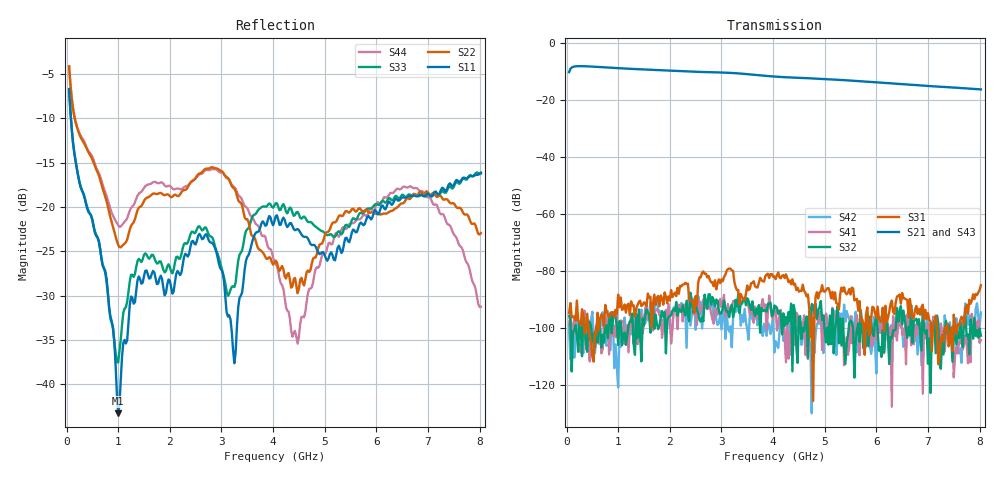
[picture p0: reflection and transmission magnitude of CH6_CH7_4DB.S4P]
!Agilent Technologies,E5071C,MY46316741,A.11.02
!Date: Mon Jun 01 10:34:16 2026
!Data & Calibration Information:
!1:CH6 INPUT 2:CH6 OUTPUT 3:CH7 INPUT 4:CH7 OUTPUT
!Freq	S11:SOLT4(ON)	S12:SOLT4(ON)	S13:SOLT4(ON)	S14:SOLT4(ON)
!	S21:SOLT4(ON)	S22:SOLT4(ON)	S23:SOLT4(ON)	S24:SOLT4(ON)
!	S31:SOLT4(ON)	S32:SOLT4(ON)	S33:SOLT4(ON)	S34:SOLT4(ON)
!	S41:SOLT4(ON)	S42:SOLT4(ON)	S43:SOLT4(ON)	S44:SOLT4(ON)
!PortZ  Port1:50+j0  Port2:50+j0  Port3:50+j0  Port4:50+j0
!Above PortZ is port z conversion or system Z0 setting when saving the data.
!When reading, reference impedance value at option line is always used.
# Hz S dB R 50
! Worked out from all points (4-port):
!   320 points, 50 MHz to 8.025 GHz, reference 50 ohm
!   strongest paths, dB at 50 MHz, 2.05 GHz, 4.05 GHz, 6.05 GHz, 8.025 GHz:
!     S21: -10.3, -9.8, -11.9, -13.9, -16.4
!     S43: -10.2, -9.8, -12.0, -14.0, -16.4
!     S31: -94.7, -89.1, -82.8, -96.9, -85.0
!     S32: -95.7, -93.9, -92.9, -107.9, -102.7
!     S41: -99.0, -100.8, -92.2, -100.9, -104.3
!     S42: -99.7, -99.6, -104.6, -101.0, -94.5
!   lowest |S11| = -43.2 dB at 1 GHz (marker M1), VSWR 1.01, Z = 49.4 - j0.283 ohm
!   |S11| at or under -10 dB: 85.48 MHz to end of sweep
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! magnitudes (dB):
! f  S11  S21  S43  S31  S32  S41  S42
! 50 MHz  -6.7  -10.3  -10.2  -94.7  -95.7  -99.0  -99.7
! 1 GHz  -43.2  -8.9  -8.9  -88.3  -105.9  -103.5  -120.8
! 2.575 GHz  -23.0  -10.2  -10.2  -82.2  -97.1  -95.2  -91.7
! 3.25 GHz  -37.6  -10.6  -10.7  -83.8  -93.9  -90.3  -94.2
! 4.475 GHz  -22.5  -12.3  -12.3  -85.8  -112.2  -95.4  -101.2
! 6.525 GHz  -18.9  -14.5  -14.6  -89.5  -93.9  -101.4  -106.5
! 8.025 GHz  -16.2  -16.4  -16.4  -85.0  -102.7  -104.3  -94.5
